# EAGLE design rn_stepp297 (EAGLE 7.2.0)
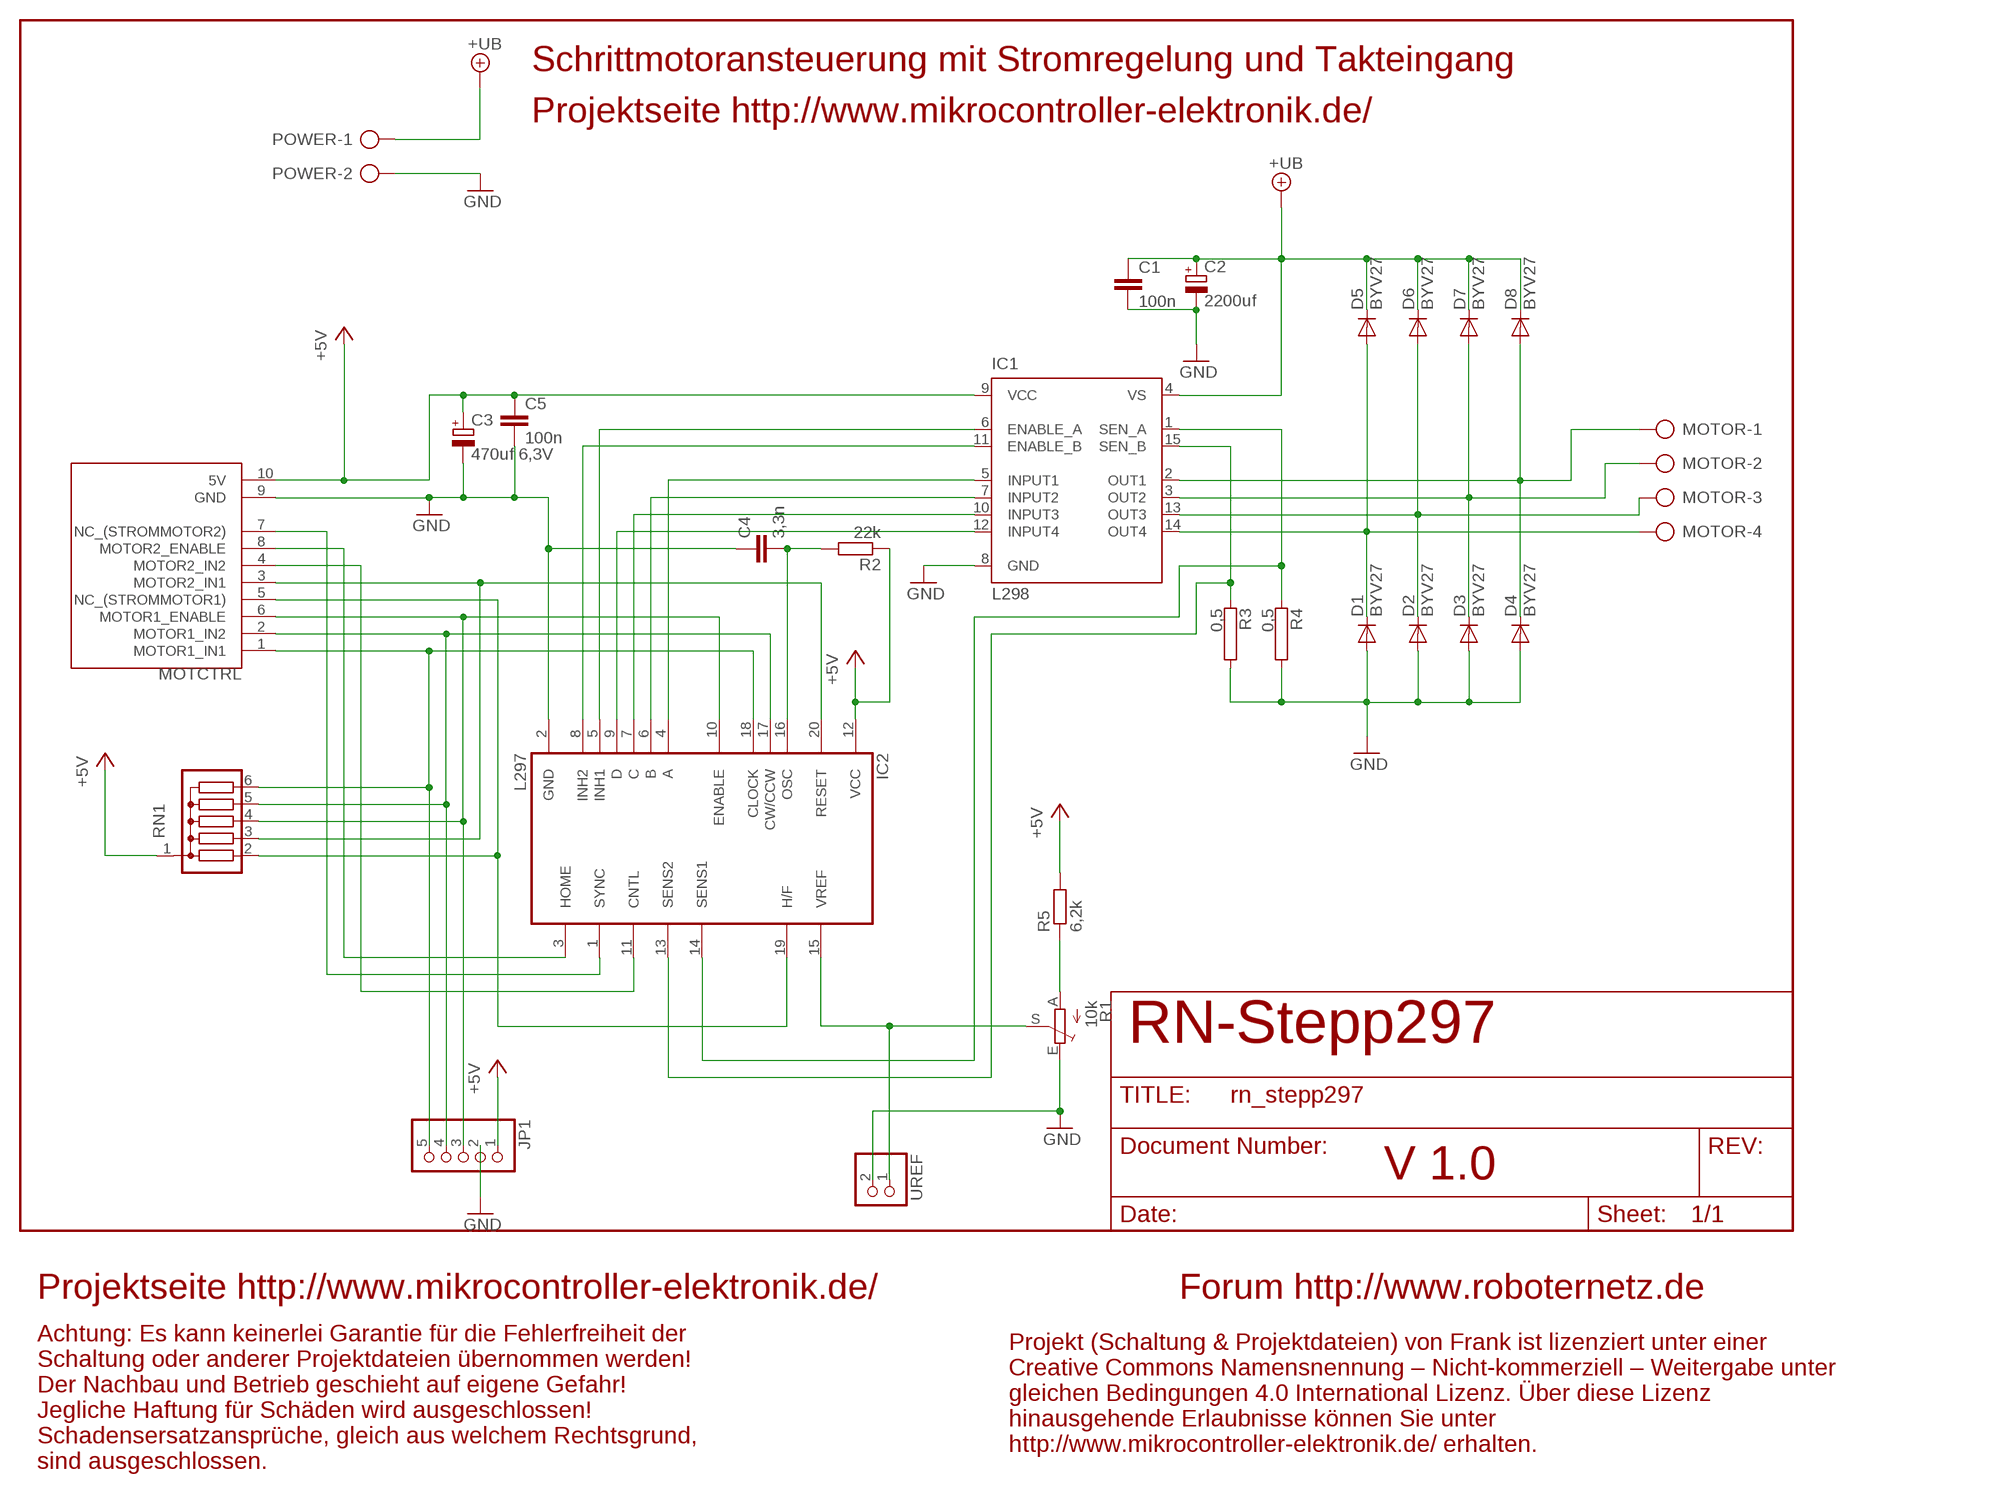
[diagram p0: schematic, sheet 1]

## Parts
C1  100n  C-EU050-024X044  [C050-024X044]
C2  2200uf  CPOL-EUE7.5-16  [E7,5-16]
C3  470uf 6,3V  CPOL-EUE3.5-8  [E3,5-8]
C4  3,3n  C-EU050-024X044  [C050-024X044]
C5  100n  C-EU050-024X044  [C050-024X044]
D1  BYV27  [SOD57-10]
D2  BYV27  [SOD57-10]
D3  BYV27  [SOD57-10]
D4  BYV27  [SOD57-10]
D5  BYV27  [SOD57-10]
D6  BYV27  [SOD57-10]
D7  BYV27  [SOD57-10]
D8  BYV27  [SOD57-10]
IC1  L298  [MULTIWATT-15]
IC2  L297  [DIL20]
JP1  PINHD-1X5  [1X05]
MOTCTRL  MOTORSTTCKER10POLRNNORM  [ML10]
MOTOR  AK220-04  [AKL220-04]
POWER  AKL220-02  [AKL220-02]
R1  10k  TRIM_EU-S64W  [S64W]
R2  22k  R-EU_0207/10  [0207/10]
R3  0,5  RKH208-8  [KH208-8]
R4  0,5  RKH208-8  [KH208-8]
R5  6,2k  R-EU_0207/10  [0207/10]
RN1  G05R  [SIL6]
UREF  PINHD-1X2  [1X02]

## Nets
+5V: C3.+ C5.1 IC1.9(VCC) IC2.12(VCC) JP1.1 MOTCTRL.10(5V) R2.1 R5.2 RN1.1
+UB [Power3A]: C1.1 C2.+ D5.C D6.C D7.C D8.C IC1.4(VS) POWER.1
GND [Power3A]: C1.2 C2.- C3.- C4.1 C5.2 D1.A D2.A D3.A D4.A IC1.8(GND) IC2.2(GND) JP1.2 MOTCTRL.9(GND) POWER.2 R1.E R3.2 R4.2 UREF.2
N$1: IC1.5(INPUT1) IC2.4(A)
N$2: IC1.7(INPUT2) IC2.6(B)
N$3: IC1.10(INPUT3) IC2.7(C)
N$4: IC1.12(INPUT4) IC2.9(D)
N$5 [Power3A]: D1.C D5.A IC1.14(OUT4) MOTOR.4
N$6 [Power3A]: D2.C D6.A IC1.13(OUT3) MOTOR.3
N$7 [Power3A]: D3.C D7.A IC1.3(OUT2) MOTOR.2
N$8 [Power3A]: D4.C D8.A IC1.2(OUT1) MOTOR.1
N$12 [Power3A]: IC1.1(SEN_A) IC2.14(SENS1) R4.1
N$18: IC2.15(VREF) R1.S UREF.1
N$19: R1.A R5.1
N$20 [Power3A]: IC1.15(SEN_B) IC2.13(SENS2) R3.1
N$24: IC2.19(H/F) MOTCTRL.5(NC_(STROMMOTOR1)) RN1.2
N$25: IC1.6(ENABLE_A) IC2.5(INH1)
N$26: IC1.11(ENABLE_B) IC2.8(INH2)
N$27: IC2.20(RESET) MOTCTRL.3(MOTOR2_IN1) RN1.3
N$28: IC2.3(HOME) MOTCTRL.8(MOTOR2_ENABLE)
N$29: C4.2 IC2.16(OSC) R2.2
N$30: IC2.1(SYNC) MOTCTRL.7(NC_(STROMMOTOR2))
N$31: IC2.11(CNTL) MOTCTRL.4(MOTOR2_IN2)
N$32: IC2.18(CLOCK) JP1.5 MOTCTRL.1(MOTOR1_IN1) RN1.6
N$33: IC2.17(CW/CCW) JP1.4 MOTCTRL.2(MOTOR1_IN2) RN1.5
N$34: IC2.10(ENABLE) JP1.3 MOTCTRL.6(MOTOR1_ENABLE) RN1.4

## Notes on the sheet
- Schrittmotoransteuerung mit Stromregelung und Takteingang
- Projektseite http://www.mikrocontroller-elektronik.de/
- RN-Stepp297
- V 1.0
- Projektseite http://www.mikrocontroller-elektronik.de/ | Forum http://www.roboternetz.de
- Projekt (Schaltung & Projektdateien) von Frank ist lizenziert unter einer
  Creative Commons Namensnennung – Nicht-kommerziell – Weitergabe unter
  gleichen Bedingungen 4.0 International Lizenz. Über diese Lizenz
  hinausgehende Erlaubnisse können Sie unter
  http://www.mikrocontroller-elektronik.de/ erhalten.
- Achtung: Es kann keinerlei Garantie für die Fehlerfreiheit der
  Schaltung oder anderer Projektdateien übernommen werden!
  Der Nachbau und Betrieb geschieht auf eigene Gefahr! 
  Jegliche Haftung für Schäden wird ausgeschlossen!
  Schadensersatzansprüche, gleich aus welchem Rechtsgrund,
  sind ausgeschlossen.

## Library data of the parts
C1 C4 C5 = rcl:C-EU: CAPACITOR, European symbol
C2 C3 = rcl:CPOL-EU: POLARIZED CAPACITOR, European symbol
D1-D8 = diode:BYV27: DIODE
IC1 = st-microelectronics:L298: DUAL FULL-BRIDGE DRIVER
IC2 = st-microelectronics:L297: STEPPER MOTOR CONTROLLER
JP1 = pinhead:PINHD-1X5: PIN HEADER
MOTCTRL = RoboterNetz:MOTORSTTCKER10POLRNNORM
MOTOR = RoboterNetz:AK220-04: CONNECTOR
POWER = RoboterNetz:AKL220-02: CONNECTOR
R1 = pot:TRIM_EU-: POTENTIOMETER
R2 R5 = rcl:R-EU_: RESISTOR, European symbol
R3 R4 = resistor-power:R: Power Resitor
RN1 = resistor-sil:G05R: SIL RESISTOR
UREF = pinhead:PINHD-1X2: PIN HEADER

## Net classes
1 Power4A: width 1.27 mm, drill 1.27 mm, clearance 0.406 mm
2 Power2A: width 0.762 mm
3 Power3A: width 1.016 mm
4 Power10A: width 1.778 mm, drill 1.778 mm, clearance 0.457 mm

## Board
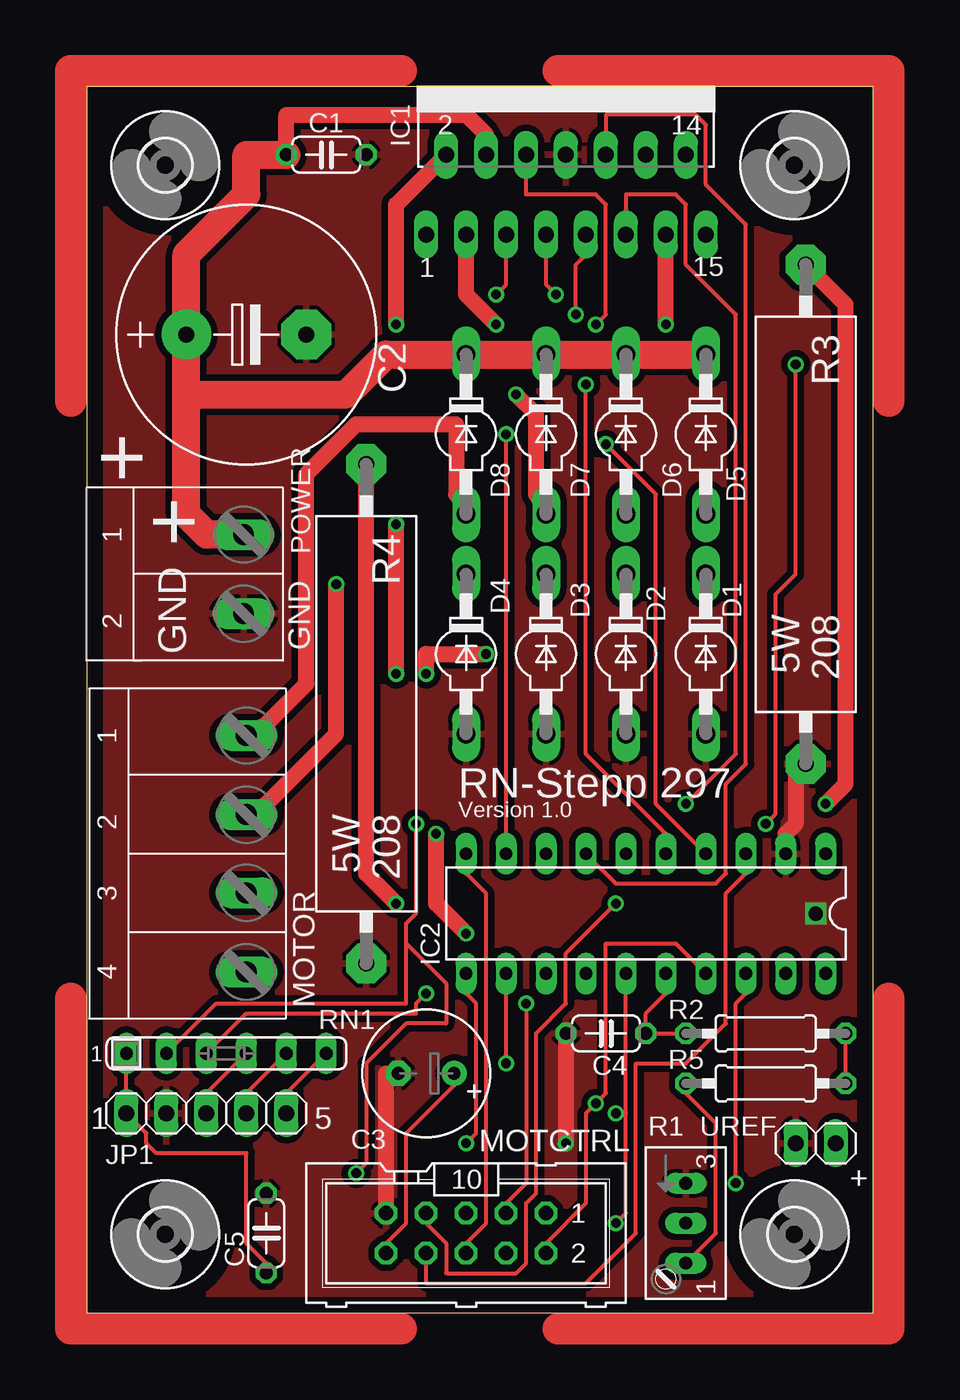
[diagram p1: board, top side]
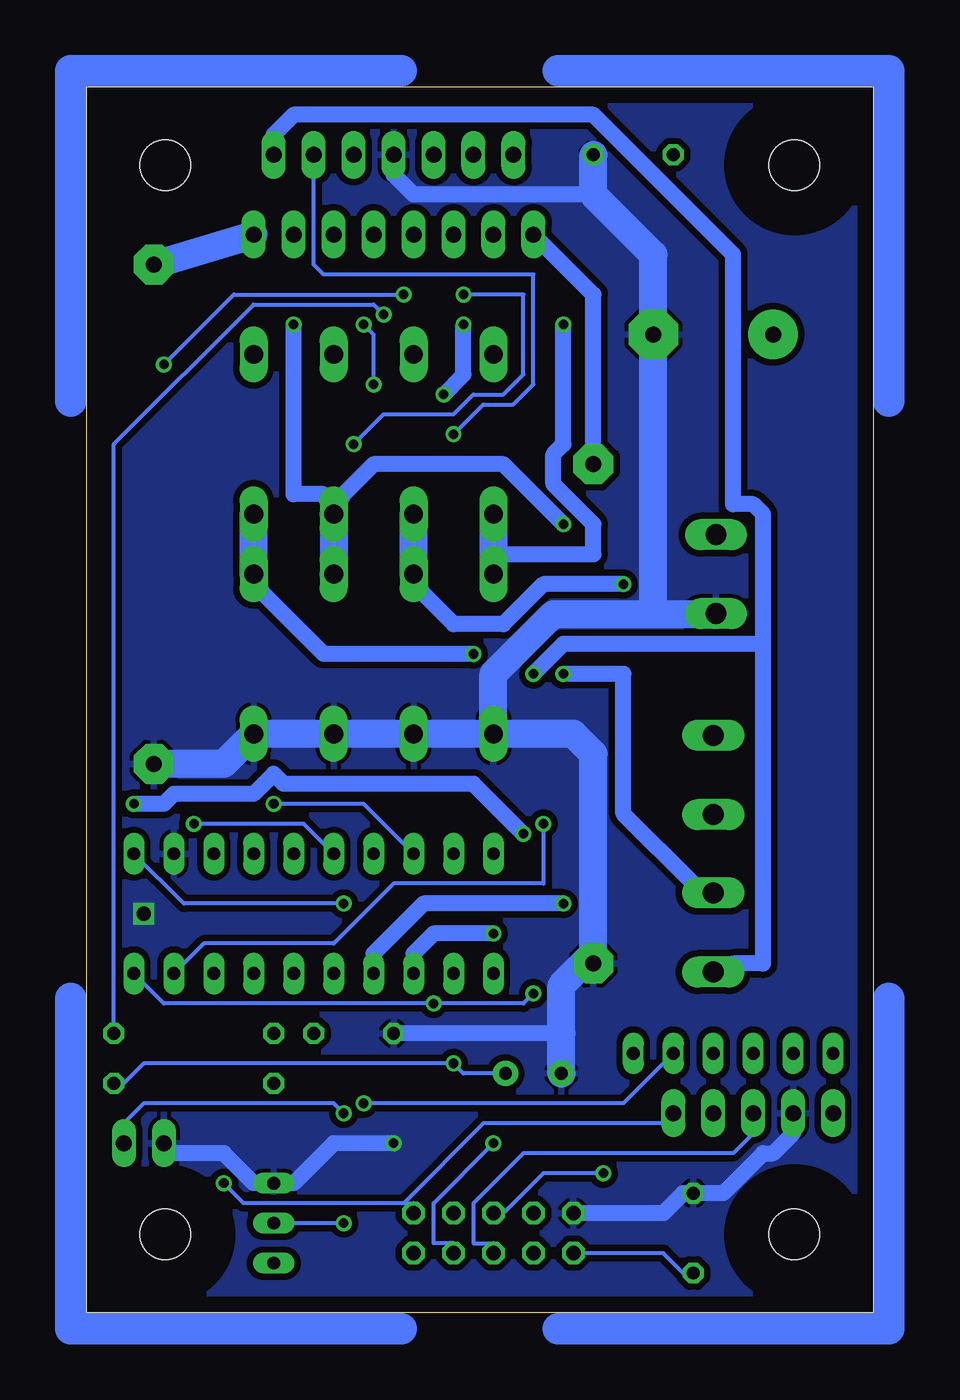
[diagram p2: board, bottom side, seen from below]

Size 50 x 78 mm. Coordinates in mm from the lower left corner, seen from the top.
Outline: 0,0 50,0 50,78 0,78 0,0
Copper layers (1*16): Top 0.035mm / dielectric 1.5mm / Bottom 0.035mm
Design rules "default": minimum track width 10mil, minimum drill 24mil, track to track 11mil, track to pad 11mil, pad to pad 11mil, via to via 11mil, smd to smd 8mil, copper to edge 40mil, drill to drill 8mil, minimum pad ring 10mil, minimum via ring 8mil, stop-mask expansion 4mil, vias tented up to drill 0mil, thermal gap 10mil

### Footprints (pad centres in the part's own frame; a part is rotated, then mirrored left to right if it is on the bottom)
C050-024X044 = drill 0.813 octagon: 1 -2.54,0; 2 2.54,0
E7,5-16 = drill 1.016 pad 3.15: + -3.81,0 | drill 1.016 pad 3.15 octagon: - 3.81,0
E3,5-8 = drill 0.813 pad 1.6: + -1.778,0 | drill 0.813 pad 1.6 octagon: - 1.778,0
SOD57-10 = drill 1.194 long: A 5.08,0; C -5.08,0
MULTIWATT-15 = drill 1.016 long: 1 -8.89,-7.62; 2 -7.62,-2.54; 3 -6.35,-7.62; 4 -5.08,-2.54; 5 -3.81,-7.62; 6 -2.54,-2.54; 7 -1.27,-7.62; 8 0,-2.54; 9 1.27,-7.62; 10 2.54,-2.54; 11 3.81,-7.62; 12 5.08,-2.54; 13 6.35,-7.62; 14 7.62,-2.54; 15 8.89,-7.62
DIL20 = drill 0.813 long: 1 -11.43,-3.81; 2 -8.89,-3.81; 3 -6.35,-3.81; 4 -3.81,-3.81; 5 -1.27,-3.81; 6 1.27,-3.81; 7 3.81,-3.81; 8 6.35,-3.81; 9 8.89,-3.81; 10 11.43,-3.81; 11 11.43,3.81; 12 8.89,3.81; 13 6.35,3.81; 14 3.81,3.81; 15 1.27,3.81; 16 -1.27,3.81; 17 -3.81,3.81; 18 -6.35,3.81; 19 -8.89,3.81; 20 -11.43,3.81
1X05 = drill 1.016 long: 1 -5.08,0; 2 -2.54,0; 3 0,0; 4 2.54,0; 5 5.08,0
ML10 = drill 0.914 octagon: 1 -5.08,-1.27; 2 -5.08,1.27; 3 -2.54,-1.27; 4 -2.54,1.27; 5 0,-1.27; 6 0,1.27; 7 2.54,-1.27; 8 2.54,1.27; 9 5.08,-1.27; 10 5.08,1.27
AKL220-04 = drill 1.321 long: 1 -7.518,2.54; 2 -2.489,2.54; 3 2.489,2.54; 4 7.518,2.54
AKL220-02 = drill 1.321 long: 1 -2.515,3; 2 2.515,3
S64W = drill 0.813 long: A 2.54,1.27; E -2.54,1.27; S 0,1.27
0207/10 = drill 0.813 octagon: 1 -5.08,0; 2 5.08,0
KH208-8 = drill 1.016 pad 2.54 octagon: 1 -15.875,0; 2 15.875,0
SIL6 = drill 0.813 long: 1 -6.35,0; 2 -3.81,0; 3 -1.27,0; 4 1.27,0; 5 3.81,0; 6 6.35,0
3,2 = hole 3.2: 0,0
1X02 = drill 1.016 long: 1 -1.27,0; 2 1.27,0

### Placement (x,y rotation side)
C1  15.24,73.66 0 top
C2  10.16,62.23 0 top
C3  21.59,15.24 180 top
C4  33.02,17.78 0 top
C5  11.43,5.08 90 top
D1  39.37,41.91 270 top
D2  34.29,41.91 270 top
D3  29.21,41.91 270 top
D4  24.13,41.91 270 top
D5  39.37,55.88 270 top
D6  34.29,55.88 270 top
D7  29.21,55.88 270 top
D8  24.13,55.88 270 top
IC1  30.48,76.2 0 top
IC2  35.56,25.4 180 top
JP1  7.62,12.7 0 top
MOTCTRL  24.13,5.08 180 top
MOTOR  7.62,29.21 270 top
POWER  6.99,46.99 270 top
R1  36.83,5.71 270 top
R2  43.18,17.78 180 top
R3  45.72,50.8 270 top
R4  17.78,38.1 270 top
R5  43.18,14.61 0 top
RN1  8.89,16.51 0 top
U$2  [3,2]  5,5 0 top
U$3  [3,2]  45,5 0 top
U$4  [3,2]  5,73 0 top
U$5  [3,2]  45,73 0 top
UREF  46.35,10.79 180 top

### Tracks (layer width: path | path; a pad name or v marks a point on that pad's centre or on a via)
+5V  (via drill 0.61)
  Top 0.254: v26.67,15.88 IC2.12 | RN1.1 JP1.1 3.81,11.43 3.81,10.79 4.45,10.16 10.16,10.16 10.16,4.45 11.43,3.17 C5.1 | C3.+ 23.5,14.61 20.32,11.43 20.32,5.71 19.05,4.45 MOTCTRL.10 | R5.2 R2.1 | v31.11,63.5 31.11,66.67 31.75,67.31 IC1.9
  Bottom 0.254: C3.+ 26.04,15.24 v26.67,15.88 46.35,15.88 47.62,14.61 R5.2 | v31.11,63.5 31.75,64.14 39.37,64.14 48.26,55.24 R2.1 | C5.1 12.06,2.54 13.34,3.81 MOTCTRL.10
+UB
  Top 1.016: IC1.4 25.4,74.93 24.13,76.2 12.7,76.2 C1.1
  Top 1.778: POWER.1 7.64,49.51 6.35,50.8 6.35,58.42 | 6.35,58.42 C2.+ 6.35,67.31 10.16,71.12 10.16,73.66 C1.1 | D5.C D6.C D7.C D8.C 19.05,60.96 16.51,58.42 6.35,58.42
GND  (via drill 0.61, 0.9)
  Top 1.016: IC2.2 44.45,30.48 45.09,31.11 45.09,34.29 R3.2 | MOTCTRL.9 19.05,15.24 C3.- | C4.1 v30.48,10.79
  Bottom 1.016: UREF.2 44.45,10.16 41.27,10.16 39.37,8.26 R1.E 36.83,8.26 34.29,10.79 v30.48,10.79 | JP1.2 5.08,11.43 6.35,10.16 6.99,10.16 9.53,7.62 C5.2 12.06,7.62 13.34,6.35 MOTCTRL.9 | 19.81,17.78 C4.1 | IC1.8 30.48,72.39 29.21,71.12 17.78,71.12
  Bottom 1.778: R3.2 41.27,34.92 D1.A D2.A D3.A D4.A | D4.A 24.13,40.64 20.32,44.45 13.97,44.45 | POWER.2 10.13,44.48 10.16,44.45 13.97,44.45 | 17.78,22.86 R4.2 | 17.78,22.86 17.78,35.56 19.05,36.83 D4.A | C3.- 19.81,17.78 19.81,20.83 17.78,22.86 | C1.2 17.78,71.12 13.97,67.31 C2.- 13.97,44.45
  other vias: 46.35,25.4
  pour Bottom (isolate 0.406): 0,0 49.53,0 49.53,77.47 0,77.47
  pour Top (isolate 0.406): 0,78.11 50.16,78.11 50.16,0 0,0 0,77.47
N$1  (via drill 0.61)
  Top 0.254: v33.02,55.24 36.2,52.07 36.2,32.38 IC2.4 | v26.04,64.77 26.67,65.41 IC1.5
  Bottom 0.254: v33.02,55.24 31.11,57.15 26.67,57.15 25.4,58.42 23.5,58.42 22.23,59.69 22.23,64.77 v26.04,64.77
N$2  (via drill 0.61)
  Top 0.254: v43.18,31.11 43.81,31.75 43.81,45.72 45.09,46.99 v45.09,60.33 | v29.84,64.77 29.21,65.41 IC1.7
  Bottom 0.254: v43.18,31.11 36.2,31.11 IC2.6 | v45.09,60.33 40.64,64.77 v29.84,64.77
N$3
  Top 0.254: IC2.7 33.66,27.3 40.01,27.3 40.64,27.94 40.64,33.66 41.91,34.92 41.91,69.22 39.37,71.75 39.37,75.56 38.73,76.2 33.02,76.2 IC1.10
N$4  (via drill 0.61)
  Top 0.254: IC2.9 v26.67,55.88
  Bottom 0.254: v26.67,55.88 24.77,57.78 22.86,57.78 21.59,59.05 21.59,66.04 34.92,66.04 35.56,66.67 IC1.12
N$5  (via drill 0.61)
  Top 1.016: v25.4,41.91 21.59,41.91 v21.59,40.64
  Bottom 1.016: 6.99,42.55 6.99,22.23 8.89,22.23 MOTOR.4 | 6.99,42.55 6.99,50.8 7.62,51.44 8.89,51.44 8.89,67.31 17.78,76.2 36.83,76.2 38.1,74.93 IC1.14 | v25.4,41.91 34.92,41.91 38.73,45.72 D1.C | v21.59,40.64 19.68,42.55 6.99,42.55
  Bottom 1.778: D1.C D5.A
N$6  (via drill 0.61)
  Top 1.016: v36.83,62.87 IC1.13 | v19.68,40.64 v19.68,50.16
  Bottom 1.016: v36.83,62.87 36.83,52.07 34.92,52.07 D6.A 33.66,52.07 31.75,53.98 23.5,53.98 v19.68,50.16 | v19.68,40.64 15.88,40.64 15.88,31.75 11.43,27.3 MOTOR.3
  Bottom 1.778: D6.A D2.C
N$7  (via drill 0.61)
  Top 1.016: v26.04,62.87 24.13,64.77 IC1.3 | v27.3,58.42 28.57,57.15 28.57,52.07 D7.A | v15.88,46.35 15.88,36.83 11.43,32.38 MOTOR.2
  Bottom 1.016: v26.04,62.87 26.04,59.69 v27.3,58.42 | v15.88,46.35 20.95,46.35 23.5,43.81 26.67,43.81 28.57,45.72 D3.C
  Bottom 1.778: D3.C D7.A
N$8  (via drill 0.61)
  Top 1.016: v19.68,62.87 19.68,70.48 IC1.2 | MOTOR.1 11.43,37.47 13.97,40.01 13.97,53.34 17.14,56.52 23.5,56.52 23.5,52.07 D8.A
  Bottom 1.016: v19.68,62.87 19.68,55.24 20.32,54.61 20.32,52.7 17.78,50.16 17.78,48.26 23.5,48.26 D4.C
  Bottom 1.778: D8.A D4.C
N$9
  Top 2: 20,-1 -1,-1 -1,20
N$10
  Top 2: 30,-1 51,-1 51,20
N$11
  Top 2: 20,79 -1,79 -1,58
N$12  (via drill 0.61)
  Top 1.016: v19.68,26.04 17.78,27.94 R4.1
  Bottom 1.016: v19.68,26.04 28.57,26.04 31.75,22.86 IC2.14 | IC1.1 17.78,64.77 R4.1
N$13
  Top 2: 51,58 51,79 30,79
N$14
  Bottom 2: 20,-1 -1,-1 -1,20
N$15
  Bottom 2: 30,-1 51,-1 51,20
N$16
  Bottom 2: 20,79 -1,79 -1,58
N$17
  Bottom 2: 51,58 51,79 30,79
N$18  (via drill 0.61)
  Top 0.254: v33.66,5.71 34.29,6.35 34.29,12.7 | 34.29,12.7 IC2.15 | 34.29,12.7 v33.66,12.7
  Bottom 0.254: v33.66,5.71 R1.S | v33.66,12.7 34.29,13.34 46.35,13.34 47.62,12.06 UREF.1
N$19
  Top 0.254: R1.A 40.01,5.08 40.01,12.06 38.1,13.97 R5.1
N$20  (via drill 0.61)
  Top 1.016: v24.13,24.13 22.23,26.04 v22.23,30.48 | v46.99,32.38 48.26,33.66 48.26,64.14 R3.1
  Bottom 1.016: v24.13,24.13 27.94,24.13 29.21,22.86 IC2.13 | v22.23,30.48 25.4,33.66 37.47,33.66 38.1,34.29 39.37,33.02 44.45,33.02 45.09,32.38 v46.99,32.38
  Bottom 1.778: R3.1 IC1.15
N$24  (via drill 0.61)
  Top 0.254: 20.32,23.5 20.32,24.77 20.95,25.4 v20.95,31.11 | 20.32,23.5 20.32,19.68 8.26,19.68 RN1.2 | v17.14,8.89 17.78,9.53 17.78,15.88 20.32,18.41 22.86,18.41 22.86,20.95 20.32,23.5
  Bottom 0.254: v20.95,31.11 20.95,27.3 30.48,27.3 34.29,23.5 42.55,23.5 IC2.19 | v17.14,8.89 20.95,8.89 23.5,6.35 MOTCTRL.5
N$25  (via drill 0.61)
  Top 0.254: v31.75,59.05 31.75,35.56 36.83,30.48 IC2.5 | v32.38,62.87 33.02,63.5 33.02,70.48 32.38,71.12 27.94,71.12 IC1.6
  Bottom 0.254: v31.75,59.05 31.75,62.23 v32.38,62.87
N$26  (via drill 0.61)
  Top 0.254: v38.1,32.38 41.27,35.56 41.27,63.5 38.1,66.67 38.1,70.48 37.47,71.12 34.29,71.12 IC1.11
  Bottom 0.254: v38.1,32.38 32.38,32.38 IC2.8
N$27  (via drill 0.61)
  Top 0.254: v21.59,20.32 20.95,19.68 20.95,19.05 10.16,19.05 RN1.3 | v27.94,19.68 27.94,8.26 26.67,6.99 MOTCTRL.3
  Bottom 0.254: v21.59,20.32 22.23,19.68 v27.94,19.68 45.09,19.68 IC2.20
N$28
  Top 0.254: IC2.3 41.91,27.94 40.64,26.67 40.64,18.41 38.1,15.88 34.92,15.88 34.92,5.08 31.75,1.91 21.59,1.91 MOTCTRL.8
N$29
  Top 0.254: R2.2 C4.2 35.56,19.05 36.83,20.32 IC2.16
N$30  (via drill 0.61)
  Top 0.254: v33.66,26.04 30.48,22.86 30.48,19.68 28.57,17.78 28.57,7.62 27.94,6.99 27.94,3.17 27.3,2.54 22.86,2.54 22.86,4.45 21.59,5.71 MOTCTRL.7
  Bottom 0.254: v33.66,26.04 43.81,26.04 IC2.1
N$31  (via drill 0.61)
  Top 0.254: v24.13,10.79 24.77,11.43 24.77,19.68 24.13,20.32 IC2.11
  Bottom 0.254: v24.13,10.79 27.94,6.99 27.94,4.45 26.67,4.45 MOTCTRL.4
N$32  (via drill 0.61)
  Top 0.254: RN1.6 12.7,13.97 JP1.5 | v41.27,8.26 41.27,19.68 41.91,20.32 IC2.18
  Bottom 0.254: v41.27,8.26 40.01,6.99 29.84,6.99 | 29.84,6.99 29.21,6.99 MOTCTRL.1 | 29.84,6.99 24.77,12.06 13.34,12.06 JP1.5
N$33  (via drill 0.61)
  Top 0.254: RN1.5 10.16,13.97 JP1.4 | IC2.17 37.47,23.5 33.02,23.5 33.02,13.97 v32.38,13.34 31.75,12.7 31.75,6.99 29.21,4.45 MOTCTRL.2
  Bottom 0.254: v32.38,13.34 15.88,13.34 RN1.5
N$34
  Top 0.254: RN1.4 7.62,13.97 JP1.3 | IC2.10 24.13,27.94 25.4,26.67 25.4,5.71 24.13,4.45 MOTCTRL.6
  Bottom 0.254: JP1.3 7.62,11.43 8.89,10.16 22.23,10.16 25.4,6.99 25.4,4.45 24.13,4.45 MOTCTRL.6

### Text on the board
tPlace: + | + | GND | GND | RN-Stepp 297 | Version 1.0 | 1 | 5 | +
